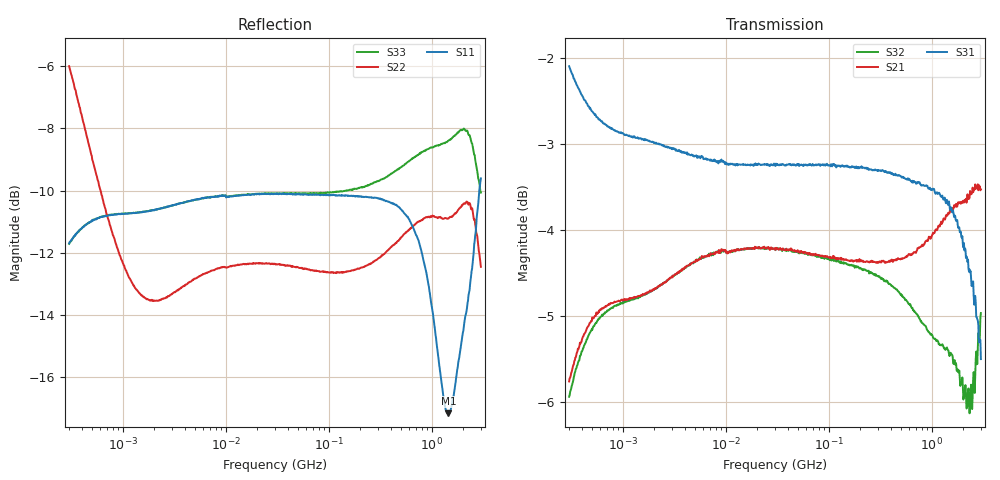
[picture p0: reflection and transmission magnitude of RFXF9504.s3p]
! RFMD Transformer
! RFXF9504 Tested 1/12/2010
! S3P Data File Format
! All S Parameters Mag in dB and Angle in Degree format
! Test Conditions: Input Power = -10dBm @ Temperature +25 deg C
! 801 Frequency points - Log Sweep
! Port 1 is Pin 1,Port 2 is Pin 4, Port 3 is Pin 3 and Pin 2 Circuit Ground.
! Frequency Mag(S11)Angle(S11)Mag(S12)Angle(S12)Mag(S13)Angle(S13)
! Mag(S21)Angle(S21)Mag(S22)Angle(S22)Mag(S23)Angle(S23)
! Mag(S31)Angle(S31)Mag(S32)Angle(S32)Mag(S33)Angle(S33)
# Hz S  dB  R 50
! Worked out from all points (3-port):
!   801 points, 300 kHz to 3 GHz, reference 50 ohm
!   strongest paths, dB at 300 kHz, 3 MHz, 30 MHz, 300 MHz, 3 GHz:
!     S31: -2.1, -3.1, -3.3, -3.3, -5.5
!     S21: -5.8, -4.5, -4.2, -4.4, -3.5
!     S32: -5.9, -4.5, -4.2, -4.5, -5.0
!   lowest |S11| = -17.2 dB at 1.453 GHz (marker M1), VSWR 1.32, Z = 39.4 - j6.55 ohm
!   |S11| at or under -10 dB: start of sweep to 2.896 GHz
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300000  -11.70 30.6  -5.94 -151.0  -2.08 -9.6
        -5.76 -149.3  -6.00 102.8  -5.77 30.6
        -2.10 -9.6  -5.94 29.0  -11.71 30.6
598578.7  -10.87 16.0  -5.02 -164.2  -2.72 -6.3
          -4.93 -163.9  -9.93 74.7  -4.94 16.1
          -2.72 -6.2  -5.02 15.9  -10.86 16.1
1503562  -10.70 7.4  -4.77 -172.5  -2.94 -3.2
         -4.76 -172.6  -13.37 45.8  -4.76 7.5
         -2.94 -3.2  -4.77 7.5  -10.69 7.5
3e7  -10.11 -1.2  -4.21 178.1  -3.25 -2.1
     -4.23 178.2  -12.36 3.1  -4.22 -0.7
     -3.25 -2.0  -4.22 -0.6  -10.10 1.1
1.629751e8  -10.17 -8.1  -4.35 169.6  -3.26 -8.5
            -4.36 169.6  -12.59 4.4  -4.40 -4.7
            -3.27 -8.5  -4.41 -4.6  -9.97 2.9
4.86543e8  -10.54 -25.2  -4.27 151.4  -3.28 -24.4
           -4.34 151.3  -11.57 9.0  -4.70 -11.4
           -3.37 -24.3  -4.73 -11.1  -9.27 4.5
9.059855e8  -12.83 -58.1  -4.04 128.4  -3.38 -45.6
            -4.12 129.0  -10.86 3.7  -5.12 -18.2
            -3.49 -45.0  -5.17 -18.1  -8.67 -3.3
1.452517e9  -17.17 -144.0  -3.84 100.6  -3.73 -73.4
            -3.80 100.6  -10.90 -7.4  -5.42 -26.8
            -3.70 -73.2  -5.40 -26.8  -8.39 -18.1
2.099526e9  -14.12 132.9  -3.65 67.5  -4.36 -109.2
            -3.65 67.9  -10.41 -18.5  -6.04 -34.0
            -4.22 -108.7  -5.89 -34.7  -8.04 -32.4
3e9  -9.61 72.6  -3.98 24.6  -6.06 -163.3
     -3.53 25.9  -12.45 -29.0  -5.08 -42.4
     -5.50 -162.2  -4.97 -42.6  -10.07 -64.8
